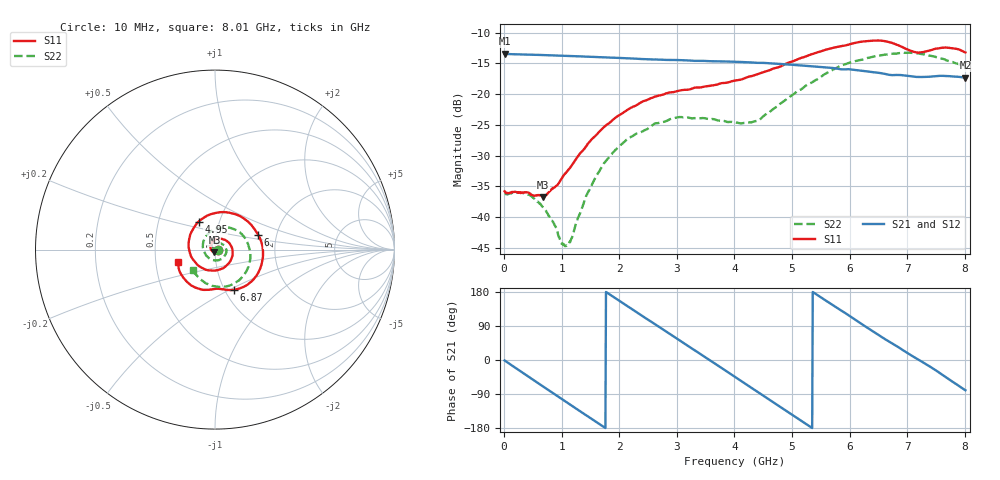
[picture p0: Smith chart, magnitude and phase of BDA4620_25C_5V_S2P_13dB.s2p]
!Agilent Technologies,E5071B,MY42404982,A.09.10
!Date: Wed May 06 09:00:54 2026
!Data & Calibration Information:
!Freq	S11:SOLT2(ON)	S21:SOLT2(ON)	S12:SOLT2(ON)	S22:SOLT2(ON)
# Hz S RI R 50
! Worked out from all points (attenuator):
!   801 points, 10 MHz to 8.01 GHz, reference 50 ohm
!   highest |S21| = -13.43 dB at 10 MHz (marker M1); lowest = -17.3 dB at 8.01 GHz (marker M2)
!   lowest |S11| = -36.7 dB at 680 MHz (marker M3), VSWR 1.03, Z = 49.7 - j1.41 ohm
!   |S11| at or under -10 dB: start of sweep to end of sweep
!   |S22| runs from -44.7 to -13.2 dB; largest |S21 - S12| = 0.00094
!   S11 on the Smith chart (normalised r, x): 10 MHz: 1.03, -0.00; 4.95 GHz: 0.80, +0.26; 6 GHz: 1.60, +0.28; 6.87 GHz: 1.10, -0.52; 8.01 GHz: 0.65, -0.10
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1e7  0.0162 -0.00116  0.2129 -0.00452  0.2132 -0.00464  0.0155 -0.00072
4.2e8  0.00897 -0.0131  0.152 -0.1442  0.1522 -0.1447  0.0136 -0.00695
6.8e8  -0.00324 -0.0142  0.0709 -0.1955  0.0709 -0.1959  0.00755 -0.00928
9.9e8  -0.0198 -0.00369  -0.0414 -0.2013  -0.0418 -0.2017  -0.00242 -0.00574
1.08e9  -0.0231 0.00162  -0.0728 -0.1915  -0.0731 -0.1918  -0.00489 -0.00325
1.16e9  -0.0245 0.00797  -0.0988 -0.1787  -0.0991 -0.1789  -0.00654 -0.000234
1.35e9  -0.0245 0.0238  -0.1511 -0.1351  -0.1513 -0.1352  -0.00862 0.00792
1.59e9  -0.0132 0.044  -0.1913 -0.0605  -0.1915 -0.0607  -0.00625 0.0201
1.9e9  0.0174 0.06  -0.1923 0.0466  -0.1926 0.0467  0.00682 0.0331
2.68e9  0.0973 -0.000699  0.00495 0.1909  0.0052 0.1913  0.0556 0.0172
3.4e9  0.0339 -0.1081  0.1786 0.0538  0.1789 0.0537  0.045 -0.0452
4.01e9  -0.0959 -0.0862  0.1305 -0.1287  0.1307 -0.129  -0.0247 -0.0537
4.41e9  -0.1461 0.00716  0.0161 -0.179  0.0159 -0.1795  -0.0602 -0.00983
4.95e9  -0.0914 0.156  -0.1323 -0.113  -0.1325 -0.1133  -0.0427 0.084
5.35e9  0.0366 0.2088  -0.1682 -0.00125  -0.1684 -0.00137  0.0311 0.1209
6e9  0.2409 0.0823  -0.0699 0.1432  -0.0701 0.1435  0.1698 0.0603
6.34e9  0.2635 -0.065  0.0213 0.1509  0.0215 0.151  0.1965 -0.0231
6.68e9  0.1782 -0.1973  0.0943 0.1085  0.0946 0.1089  0.1775 -0.1151
6.87e9  0.1031 -0.2239  0.1221 0.0748  0.1224 0.075  0.1464 -0.1586
7.19e9  0.0145 -0.2173  0.1378 0.00307  0.1382 0.00325  0.0627 -0.2053
7.56e9  -0.0956 -0.2162  0.117 -0.0784  0.1174 -0.0784  -0.0394 -0.1924
8.01e9  -0.2063 -0.0715  0.0239 -0.134  0.024 -0.1342  -0.1249 -0.1115
